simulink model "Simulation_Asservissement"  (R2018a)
settings: Solver=VariableStepAuto  StartTime=0.0  StopTime=10.0  RelTol=1e-3
libraries: fl_lib x9, nesl_utility x3, elec_lib x1, simulink x1

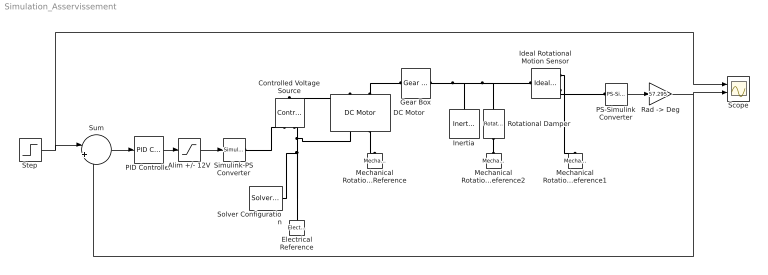
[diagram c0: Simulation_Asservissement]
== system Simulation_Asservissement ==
  Alim +/- 12V : Saturate  UpperLimit=12  LowerLimit=-12
  Controlled Voltage Source : fl_lib/Electrical/Electrical Sources/Controlled Voltage Source
  DC Motor : elec_lib/Actuators & Drivers/Rotational Actuators/DC Motor  parameterization=1  Ra=r_induit Ohm  La=1.2e-5 H  emf_or_torque=1  Kv=k V/(rad/s)  Ki=6.876e-4 N*m/A  T_stall=2.4e-4 N*m  w_max=1.91e+4 rpm  w_rated=1.5e+4 rpm  P_rated=0.08 W  V_rated=1.5 V  J=0 kg*m^2  lam_param=1  lam=0 N*m/(rad/s)  i_noload=0 A  V_i_noload=1.5 V  speed0=0 rpm  alpha=0.00393 1/K  Tmeas=25 degC  thermal_mass=100 J/K  initial_temperature=25 degC
  Electrical Reference : fl_lib/Electrical/Electrical Elements/Electrical Reference
  Gear Box : fl_lib/Mechanical/Mechanisms/Gear Box  ratio=r1  t_in_specify=off  t_in_priority=None  t_in=0 N*m  t_in_nominal_specify=off  t_in_nominal_unit=N*m  t_in_nominal_value=1  t_out_specify=off  t_out_priority=None  t_out=0 N*m  t_out_nominal_specify=off  t_out_nominal_unit=N*m  t_out_nominal_value=1
  Ideal Rotational Motion Sensor : fl_lib/Mechanical/Mechanical Sensors/Ideal Rotational Motion Sensor  offset=0 rad
  Inertia : fl_lib/Mechanical/Rotational Elements/Inertia  inertia=0.000005 kg*m^2  w_specify=off  w_priority=High  w=0 rad/s  w_nominal_specify=off  w_nominal_unit=rad/s  w_nominal_value=1  t_specify=off  t_priority=None  t=0 N*m  t_nominal_specify=off  t_nominal_unit=N*m  t_nominal_value=1
  Mechanical Rotational Reference : fl_lib/Mechanical/Rotational Elements/Mechanical Rotational Reference
  Mechanical Rotational Reference1 : fl_lib/Mechanical/Rotational Elements/Mechanical Rotational Reference
  Mechanical Rotational Reference2 : fl_lib/Mechanical/Rotational Elements/Mechanical Rotational Reference
  PID Controller : simulink/Continuous/PID Controller  Controller=PID  TimeDomain=Continuous-time  SampleTime=-1  IntegratorMethod=Forward Euler  FilterMethod=Forward Euler  Form=Parallel  UseFilter=on  ControllerParametersSource=internal  P=1  I=0  D=0  N=100  InitialConditionSource=internal  InitialConditionForIntegrator=0  InitialConditionForFilter=0  ExternalReset=none  LimitOutput=off  UpperSaturationLimit=inf  LowerSaturationLimit=-inf  LinearizeAsGain=on  AntiWindupMode=none  Kb=1  TrackingMode=off  Kt=1  PParamMin=[]  PParamMax=[]  IParamMin=[]  IParamMax=[]  DParamMin=[]  DParamMax=[]  NParamMin=[]  NParamMax=[]  KbParamMin=[]  KbParamMax=[]  KtParamMin=[]  KtParamMax=[]  POutMin=[]  POutMax=[]  IOutMin=[]  IOutMax=[]  DOutMin=[]  DOutMax=[]  NOutMin=[]  NOutMax=[]  KbOutMin=[]  KbOutMax=[]  KtOutMin=[]  KtOutMax=[]  IntegratorOutMin=[]  IntegratorOutMax=[]  FilterOutMin=[]  FilterOutMax=[]  SumOutMin=[]  SumOutMax=[]  SumI1OutMin=[]  SumI1OutMax=[]  SumI2OutMin=[]  SumI2OutMax=[]  SumI3OutMin=[]  SumI3OutMax=[]  SumDOutMin=[]  SumDOutMax=[]  SaturationOutMin=[]  SaturationOutMax=[]  IntegratorContinuousStateAttributes=''  IntegratorStateMustResolveToSignalObject=off  IntegratorRTWStateStorageClass=Auto  FilterContinuousStateAttributes=''  FilterStateMustResolveToSignalObject=off  FilterRTWStateStorageClass=Auto  DifferentiatorICPrevScaledInput=0  DifferentiatorOutMin=[]  DifferentiatorOutMax=[]  InitialConditionSetting=State (most efficient)  FilterDiffOutCoefMin=[]  FilterDiffOutCoefMax=[]  SumDenOutMin=[]  SumDenOutMax=[]  SumNumOutMin=[]  SumNumOutMax=[]  ReciprocalOutMin=[]  ReciprocalOutMax=[]  DivideOutMin=[]  DivideOutMax=[]  TunerSelectOption=Transfer Function Based (PID Tuner App)
  PS-Simulink Converter : nesl_utility/PS-Simulink Converter  PhysicalDomain=network_engine_domain  SubClassName=ps_output  LeftPortType=input  RightPortType=output  PseudoPeriodic=off  Frequencies=[]  Unit=1  AffineConversion=off
  "Rad -> Deg" : Gain  Gain=57.295
  Rotational Damper : fl_lib/Mechanical/Rotational Elements/Rotational Damper  D=0.00003 N*m/(rad/s)  w_specify=off  w_priority=None  w=0 rad/s  w_nominal_specify=off  w_nominal_unit=rad/s  w_nominal_value=1  t_specify=off  t_priority=None  t=0 N*m  t_nominal_specify=off  t_nominal_unit=N*m  t_nominal_value=1
  Scope : Scope  NumInputPorts=2
  Simulink-PS Converter : nesl_utility/Simulink-PS Converter  PhysicalDomain=network_engine_domain  SubClassName=ps_input  LeftPortType=input  RightPortType=output  PseudoPeriodic=off  Frequencies=[]  NoiseDistribution=none  NoiseParameters=[]  Unit=1  AffineConversion=off  FilteringAndDerivatives=provide  SimscapeFilterOrder=1  InputFilterTimeConstant=0.001  UdotUserProvided=0
  Solver Configuration : nesl_utility/Solver Configuration  PhysicalDomain=network_engine_domain  SubClassName=solver  LeftPortType=input  RightPortType=generic  Tones=[]  Harmonics=[]  SimulateNoise=off  Profile=off  UseLocalSampling=off  EnableSwitchedLinearOptims=on  FrequencyDomain=off  UseCCode=off  RelTol=0.001  AbsTol=1e-06  MinStep=1e-09  ToWorkspace=off  RevertToSquareIcSolve=off  NumHomotopyIterations=100  PhasorMode=off  PhasorModeNumHarmonics=1  DoDC=off  ResidualTolerance=1e-09  UseLocalSolver=off  LocalSolverChoice=NE_BACKWARD_EULER_ADVANCER  LocalSolverSampleTime=0.001  DoFixedCost=off  MaxNonlinIter=3  MaxModeIter=2  LinearAlgebra=Sparse  EquationFormulation=NE_TIME_EF  DelaysMemoryBudget=1024  AutomaticFiltering=on  FilteringTimeConstant=0.001
  Step : Step  Time=2  After=45  SampleTime=0
  Sum : Sum  Inputs=|+-
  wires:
  Alim +/- 12V/1 -> Simulink-PS Converter/1
  PS-Simulink Converter/1 -> "Rad -> Deg"/1
  PID Controller/1 -> Alim +/- 12V/1
  Sum/1 -> PID Controller/1
  Step/1 -> Scope/1, Sum/1
  "Rad -> Deg"/1 -> Scope/2, Sum/2
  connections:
  DC Motor/LConn1 -- Controlled Voltage Source/LConn1
  Controlled Voltage Source/RConn2 -- DC Motor/RConn1 -- Electrical Reference/LConn1 -- Solver Configuration/RConn1
  DC Motor/RConn2 -- Mechanical Rotational Reference/LConn1
  DC Motor/LConn2 -- Gear Box/LConn1
  Gear Box/RConn1 -- Inertia/LConn1 -- Rotational Damper/LConn1 -- Ideal Rotational Motion Sensor/LConn1
  Ideal Rotational Motion Sensor/RConn1 -- Mechanical Rotational Reference1/LConn1
  Ideal Rotational Motion Sensor/RConn3 -- PS-Simulink Converter/LConn1
  Simulink-PS Converter/RConn1 -- Controlled Voltage Source/RConn1
  Mechanical Rotational Reference2/LConn1 -- Rotational Damper/RConn1
